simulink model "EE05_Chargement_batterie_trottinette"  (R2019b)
settings: Solver=ode15s  StartTime=0.0  StopTime=14400  RelTol=1e-3  EnableMultiTasking=on
undefined symbols (not defined in the file): Ion, Lithium
libraries: electricdrivelib x2, powerlib x2

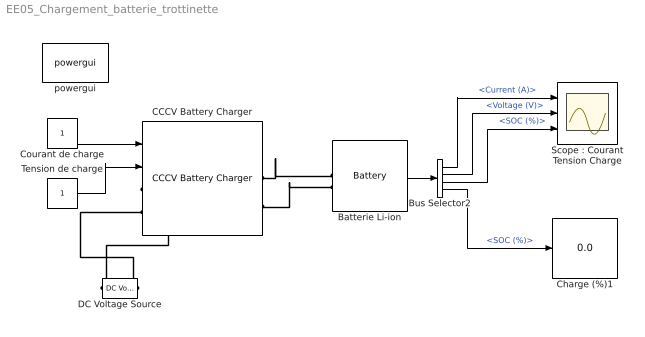
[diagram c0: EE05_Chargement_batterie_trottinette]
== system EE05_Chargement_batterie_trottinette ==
  Batterie Li-ion : electricdrivelib/Extra Sources/Battery  BatType=Lithium-Ion  ShowTempParam=off  ThermalPreset=no  ShowAgeParam=off  NomV=1  NomQ=1  SOC=1  Batt_Tr=1  PresetModel=on  MaxQ=1  MinV=0.75  FullV=1.164  Dis_rate=0.43478  R=0.01  Normal_OP=0.90435  expZone="[1.0804     0.04913]"  current=[1.5 3]  Units=Ampere-hour  Tci=20  NomT=20  T2=-30  MaxQ2=4.8  FullV2=7.1  Normal_OP2=5.655  expZone2="[6.58           1]"  Rca=0.6  ti=2000  Dp=0  Neq0=0  Tsim=1e6  Ta1=25  Qeol=5.4*0.9  Reol=0.013333*1.2  Char_age=[2.3478, 3]  Dis_age=[2.3478, 10]  N1=1500  N2=10500  N3=1000  N4=1400  Ta2=45  N5=950
  Bus Selector2 : BusSelector  OutputSignals=Current (A),Voltage (V),SOC (%),SOC (%)
  CCCV Battery Charger : electricdrivelib/Extra Sources/CCCV Battery Charger  Preset=Custom specifications  P_nom=100  s_type=DC  n_connect=off  eff_volt=230  in_freq=50  in_I_ripple=10  in_I_freq=1000  EFF_en=off  EFF_val=[0.627 0.803 0.855 0.871 0.872 0.864]  EFF_fu=[0.063 0.177 0.293 0.483 0.674 0.914]  THD_en=off  I_THD_val=[0.327 0.394 0.394 0.351 0.289 0.265]  I_THD_fu=[0.056 0.136 0.194 0.303 0.555 0.916]  H_DIST_rt=[0.199 1.297 0.328 0.029 0.416 0.200]  H_DIST_fr=[3 5 7 9 11 13]  PF_en=off  PF_val=[0.316 0.532 0.662 0.731 0.780 0.792]  PF_fu=[0.067 0.230 0.445 0.625 0.794 0.919]  Out_mode=Constant Current - Constant Voltage (CCCV)  DynInT=on  I_cst=0.1  V_cst=2.5  ABS_en=off  V_abs=142  ABS_end=Time based  ABS_time=3600  ABS_i=40  ripple=0.5  swF=1000  overshoot=1  stable_t=5  VoltComp=off  V_comp=-0.18  nom_temp=20
  Charge (%)1 : Display
  Courant de charge : Constant
  DC Voltage Source : powerlib/Electrical Sources/DC Voltage Source  Amplitude=230  Measurements=None
  "Scope : Courant Tension Charge" : Scope  NumInputPorts=3
  Tension de charge : Constant
  powergui : powerlib/powergui  Priority=1  SimulationMode=Continuous  SampleTime=50e-6  frequency=50  Iterations=50  frequencyindice=0  Pbase=100e6  ErrMax=1e-4  UnitsV=kV  UnitsW=MW  buscounter=0  FunctionMessages=off  echomessages=off  EnableUseOfTLC=off  CurrentSourceSwitches=on  DisableSnubberDevices=off  DisableRonSwitches=off  DisableVfSwitches=off  DisplayEquations=off  AutomaticDiscreteSolvers=off  SolverType=Tustin/Backward Euler (TBE)  Interpol=off  ExternalGateDelay=off  methode=off  Ts=100  x0status=blocks  SPID=off  SwTol=0  HookPort=off  NonlinearTolerance=1e-4  nMaxIteration=100  ContinueOnMaxIteration=off  RestoreLinks=warning  ResistiveCurrentMeasurement=off  Frange=[0:2:500]  Ylog=off  Xlog=on  ShowGrid=off  save=off  variable=ZData  structure=0  ZoomFFT=off  StartTime=0.0  cycles=1  DisplayStyle=1  fundamental=60  FreqAxis=off  MaxFrequency=1000  frequencyindicesteady=1  RmsSteady=1  display=off
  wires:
  Batterie Li-ion/1 -> Bus Selector2/1
  Courant de charge/1 -> CCCV Battery Charger/1
  Tension de charge/1 -> CCCV Battery Charger/2
  Bus Selector2/1 -> "Scope : Courant Tension Charge"/1  "<Current (A)>"
  Bus Selector2/2 -> "Scope : Courant Tension Charge"/2  "<Voltage (V)>"
  Bus Selector2/3 -> "Scope : Courant Tension Charge"/3  "<SOC (%)>"
  Bus Selector2/4 -> Charge (%)1/1  "<SOC (%)>"
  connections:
  CCCV Battery Charger/RConn2 -- Batterie Li-ion/LConn2
  CCCV Battery Charger/RConn1 -- Batterie Li-ion/LConn1
  DC Voltage Source/RConn1 -- CCCV Battery Charger/LConn1
  DC Voltage Source/LConn1 -- CCCV Battery Charger/LConn2
